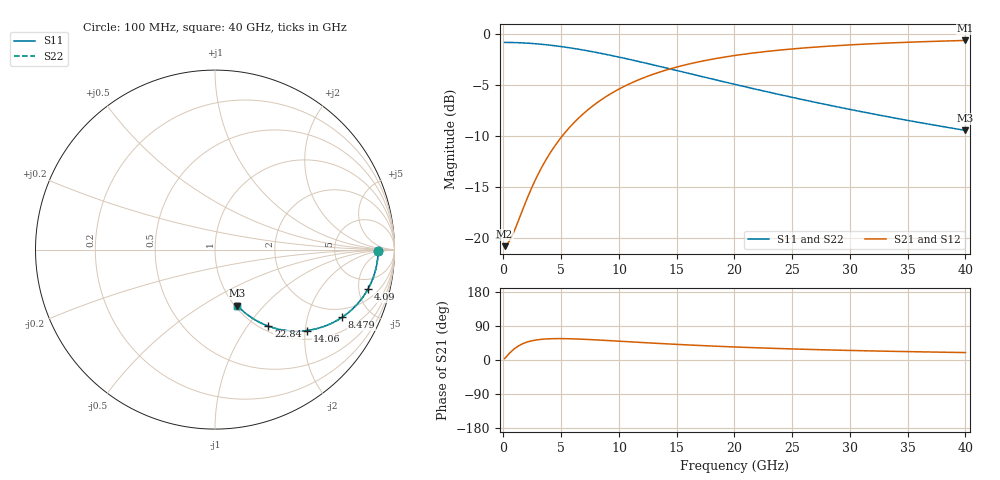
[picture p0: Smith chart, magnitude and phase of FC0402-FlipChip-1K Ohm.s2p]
!Vishay Thin-Film
!FC Family
!Case Size 0402
!Assembly Style Flip-Chip
!10/21/2015
!thinfilm@vishay.com
# GHz S MA R 50
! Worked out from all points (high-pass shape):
!   101 points, 100 MHz to 40 GHz, reference 50 ohm
!   highest |S21| = -0.63 dB at 40 GHz (marker M1); lowest = -20.8 dB at 100 MHz (marker M2)
!   |S21| within 3 dB of the highest: 13.81 GHz to end of sweep
!   lowest |S11| = -9.5 dB at 40 GHz (marker M3), VSWR 2.02, Z = 51.3 - j36.2 ohm
!   |S11| at or under -10 dB: nowhere
!   |S22| runs from -9.5 to -0.8 dB; largest |S21 - S12| = 0
!   S11 on the Smith chart (normalised r, x): 100 MHz: 21, -1; 4.09 GHz: 3.23, -6.30; 8.479 GHz: 1.57, -3.32; 14.06 GHz: 1.21, -2.04; 22.84 GHz: 1.08, -1.26; 40 GHz: 1.03, -0.72
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0.1  0.9091 -0.4  0.09112 3.6  0.09112 3.6  0.9091 -0.4
0.499  0.9086 -1.8  0.09609 17.2  0.09609 17.2  0.9086 -1.8
0.898  0.9077 -3.2  0.1068 28.5  0.1068 28.5  0.9077 -3.2
2.095  0.9014 -7.5  0.1584 47.8  0.1584 47.8  0.9014 -7.5
2.494  0.8982 -8.9  0.1787 50.9  0.1787 50.9  0.8982 -8.9
3.292  0.8903 -11.7  0.2209 54.6  0.2209 54.6  0.8903 -11.7
4.09  0.8806 -14.4  0.2635 56.1  0.2635 56.1  0.8806 -14.4
5.287  0.8629 -18.3  0.3262 56.3  0.3262 56.3  0.8629 -18.3
6.085  0.8494 -20.9  0.3664 55.7  0.3664 55.7  0.8494 -20.9
6.883  0.8347 -23.3  0.4049 54.8  0.4049 54.8  0.8347 -23.3
8.479  0.8027 -28.0  0.4762 52.3  0.4762 52.3  0.8027 -28.0
9.676  0.7773 -31.2  0.5244 50.2  0.5244 50.2  0.7773 -31.2
10.873  0.7512 -34.3  0.5682 48.1  0.5682 48.1  0.7512 -34.3
13.666  0.6904 -40.6  0.6543 43.4  0.6543 43.4  0.6904 -40.6
14.065  0.6819 -41.4  0.6649 42.7  0.6649 42.7  0.6819 -41.4
16.858  0.6248 -46.6  0.7291 38.5  0.7291 38.5  0.6248 -46.6
20.05  0.566 -51.5  0.7846 34.4  0.7846 34.4  0.566 -51.5
22.843  0.5205 -55.1  0.8216 31.3  0.8216 31.3  0.5205 -55.1
26.833  0.4646 -59.3  0.8609 27.6  0.8609 27.6  0.4646 -59.3
30.025  0.4265 -62.0  0.8842 25.2  0.8842 25.2  0.4265 -62.0
33.616  0.3898 -64.6  0.9043 22.9  0.9043 22.9  0.3898 -64.6
40  0.3368 -68.3  0.9295 19.7  0.9295 19.7  0.3368 -68.3
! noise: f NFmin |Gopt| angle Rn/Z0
0.1  -7.232e-15  1  -1.207e-06  19.91
4.489  1.929e-15  1  -1.207e-06  1.89
8.878  4.756e-08  1  0  0.5197
13.27  0  1  -8.538e-07  0.236
17.66  0  1  1.607e-14  0.1339
22.05  0  1  -7.007e-15  0.08607
26.43  5.483e-09  1  9.025e-15  0.05991
30.82  0  1  -8.559e-15  0.04407
35.21  0  1  -8.538e-07  0.03376
40  0  1  -1.479e-06  0.02615
